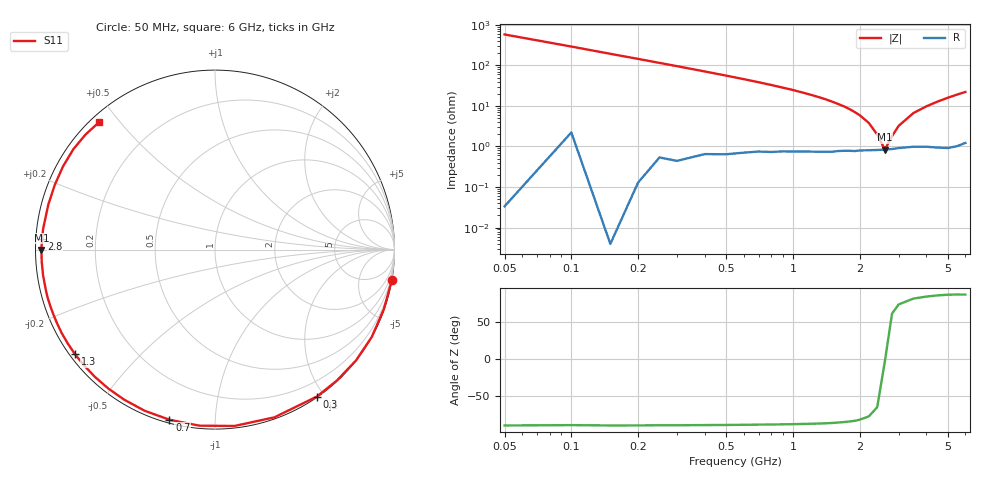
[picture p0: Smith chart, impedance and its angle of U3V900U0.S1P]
! SIEMENS Discrete & RF Semiconductors
! BBY53-02W
! Si Tuning Diode in SCD-80
! VR = 0.9 V
! S-Parameters:  September  1997
# GHz  S  MA  R  50
!  f  S11
! GHz  MAG  ANG
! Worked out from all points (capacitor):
!   34 points, 50 MHz to 6 GHz, reference 50 ohm
!   read as one part to ground: C = 5.49 pF near 50 MHz
!   lowest |Z| = 837 mohm at 2.6 GHz (marker M1)
!   series resonance near 2.605 GHz, so ESL is about 680 pH
!   S11 on the Smith chart (normalised r, x): 50 MHz: 0, -12; 300 MHz: 0.01, -1.91; 700 MHz: 0.02, -0.77; 1.3 GHz: 0.01, -0.33; 2.8 GHz: 0.02, +0.03; 6 GHz: 0.02, +0.44
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0.05  1 -9.9
0.1  0.9975 -19.5
0.15  1 -29.1
0.2  0.9994 -38.2
0.25  0.9966 -47.0
0.3  0.9962 -55.3
0.4  0.9914 -70.5
0.5  0.9886 -83.7
0.6  0.9848 -95.1
0.7  0.9813 -105.0
0.8  0.9797 -113.6
0.9  0.9773 -121.1
1  0.976 -127.5
1.1  0.9748 -133.4
1.2  0.9742 -138.6
1.3  0.9736 -143.2
1.5  0.9725 -151.3
1.6  0.971 -154.9
1.9  0.9702 -164.0
2.4  0.9678 -175.9
2.6  0.9671 -179.9
2.8  0.9659 176.4
3.5  0.962 164.9
4  0.9627 158.0
4.5  0.9654 151.3
5  0.9673 144.7
5.5  0.965 138.4
6  0.9598 132.4
